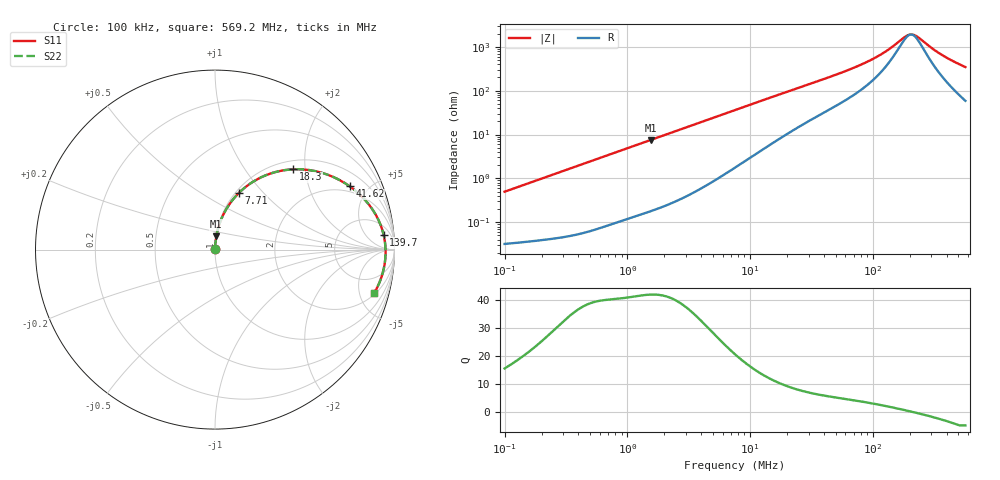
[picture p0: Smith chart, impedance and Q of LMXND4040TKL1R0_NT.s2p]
! LMXND4040TKL1R0_NT  S-PARAMETER MODEL  ( Standard Model )
! Model Generated by TAIYO YUDEN Corporation (https://www.yuden.co.jp/en/)
! Version 1.0
! TAIYO YUDEN Control No. 20250409
! Copyright(c) 2025 TAIYO YUDEN CO.,LTD. All Rights Reserved.
! Product Description (link to TY-COMPAS)
! https://ds.yuden.co.jp/TYCOMPAS/or/detail?pn=LMXND4040TKL1R0NNT&u=M
! Products Name : Inductors
! Characteristics :
!  Inductance : 1.0 [uH] , SRF(min) : 90 [MHz] , DC Resistance(max) : 0.0324 [Ohm]
!  Rated Current : Saturation  4000 [mA] , Temp Rise  3500 [mA] (40 [degC])
!  Case Size : 4.0 x 4.0 / 0.157 x 0.157 [mm/inch] , Thickness : 1.8 / 0.071 [mm/inch]
!  (Conditions: Temperature = 25 [degC] , DC Bias Current = 0 [A])
! External Node Assignments :
!  1  o---GGG---o  2
! GND o---------o GND
! Frequency Range : 0.1MHz  -  569.217162MHz  [ 402 STEP ]
# MHz S RI R 50
! Freq[MHz].  S11 Real  S11 Imag  S21 Real  S21 Imag  S12 Real  S12 Imag  S22 Real  S22 Imag
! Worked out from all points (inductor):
!   401 points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, 100 kHz to 569.2 MHz, reference 50 ohm
!   read as one part in series: L = 787 nH near 104.4 kHz
!   highest Q = 42 at 1.557 MHz (marker M1), where L = 770 nH
!   self-resonance near 204.8 MHz
!   S11 on the Smith chart (normalised r, x): 100 kHz: 1.00, +0.01; 7.71 MHz: 1.04, +0.74; 18.3 MHz: 1.18, +1.72; 41.62 MHz: 1.67, +3.77; 139.7 MHz: 11, +16; 569.2 MHz: 2.17, -6.81
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0.1  0.000345 0.00496  0.9997 -0.00496  0.9997 -0.00496  0.000345 0.00496
0.425607  0.000991 0.0208  0.999 -0.0208  0.999 -0.0208  0.000991 0.0208
1.557044  0.0074 0.0746  0.9926 -0.0746  0.9926 -0.0746  0.0074 0.0746
1.811416  0.00964 0.0865  0.9904 -0.0865  0.9904 -0.0865  0.00964 0.0865
4.208795  0.045 0.1921  0.955 -0.1921  0.955 -0.1921  0.045 0.1921
7.709517  0.132 0.3147  0.868 -0.3147  0.868 -0.3147  0.132 0.3147
11.37666  0.2425 0.3956  0.7575 -0.3956  0.7575 -0.3956  0.2425 0.3956
18.30438  0.4342 0.4472  0.5658 -0.4472  0.5658 -0.4472  0.4342 0.4472
32.11057  0.6653 0.4018  0.3347 -0.4018  0.3347 -0.4018  0.6653 0.4018
41.62041  0.7498 0.3531  0.2502 -0.3531  0.2502 -0.3531  0.7498 0.3531
60.10432  0.8402 0.2719  0.1598 -0.2719  0.1598 -0.2719  0.8402 0.2719
83.12442  0.894 0.1969  0.106 -0.1969  0.106 -0.1969  0.894 0.1969
107.7425  0.9222 0.1381  0.0778 -0.1381  0.0778 -0.1381  0.9222 0.1381
136.6649  0.9387 0.0859  0.0613 -0.0859  0.0613 -0.0859  0.9387 0.0859
139.6514  0.9398 0.0813  0.0602 -0.0813  0.0602 -0.0813  0.9398 0.0813
189.0079  0.9494 0.017  0.0506 -0.017  0.0506 -0.017  0.9494 0.017
201.6715  0.9502 0.00325  0.0498 -0.00325  0.0498 -0.00325  0.9502 0.00325
215.1836  0.9504 -0.0105  0.0496 0.0105  0.0496 0.0105  0.9504 -0.0105
234.6184  0.9501 -0.0289  0.0499 0.0289  0.0499 0.0289  0.9501 -0.0289
361.5146  0.9356 -0.1258  0.0644 0.1258  0.0644 0.1258  0.9356 -0.1258
458.5599  0.9158 -0.1844  0.0842 0.1844  0.0842 0.1844  0.9158 -0.1844
569.2172  0.8875 -0.2414  0.1125 0.2414  0.1125 0.2414  0.8875 -0.2414
